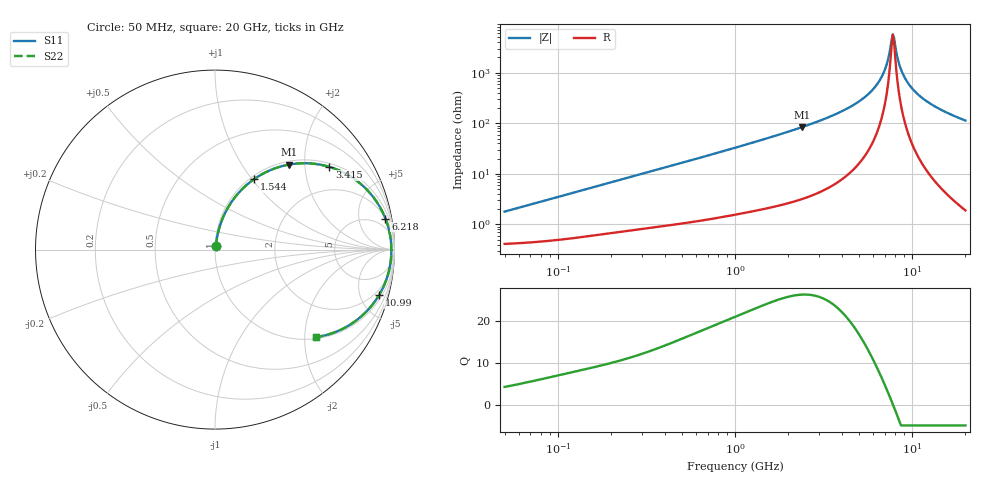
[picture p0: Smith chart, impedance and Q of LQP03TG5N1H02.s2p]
!Murata Part Number: LQP03TG5N1H02
!These Parameters are Measured in Series Mode Connection
!  o--[Z]--o
!Port1  Port2
!  o-------o
!Freq. Start=50[MHz] Stop=20[GHz], 401[Steps]
# Hz S RI R 50
!Freq.(Hz) S11(Real) S11(Imag) S21(Real) S21(Imag) S12(Real) S12(Imag) S22(Real) S22(Imag)
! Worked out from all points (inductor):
!   401 points, 50 MHz to 20 GHz, reference 50 ohm
!   read as one part in series: L = 5.55 nH near 51.52 MHz
!   highest Q = 26.4 at 2.384 GHz (marker M1), where L = 5.58 nH
!   self-resonance near 7.784 GHz
!   S11 on the Smith chart (normalised r, x): 50 MHz: 1.01, +0.03; 1.544 GHz: 1.04, +1.03; 3.415 GHz: 1.11, +2.68; 6.218 GHz: 2, +11; 10.99 GHz: 1.40, -7.03; 20 GHz: 1.04, -2.27
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5e7  0.00441 0.0173  0.9956 -0.0173  0.9956 -0.0173  0.00441 0.0173
1.364002e8  0.00775 0.0461  0.9922 -0.0461  0.9922 -0.0461  0.00775 0.0461
3.721004e8  0.0235 0.1192  0.9765 -0.1192  0.9765 -0.1192  0.0235 0.1192
1e9  0.1081 0.2877  0.8919 -0.2877  0.8919 -0.2877  0.1081 0.2877
1.544007e9  0.2184 0.3931  0.7816 -0.3931  0.7816 -0.3931  0.2184 0.3931
2.383959e9  0.4145 0.4741  0.5855 -0.4741  0.5855 -0.4741  0.4145 0.4741
2.728004e9  0.4936 0.4813  0.5064 -0.4813  0.5064 -0.4813  0.4936 0.4813
3.415248e9  0.6367 0.4611  0.3633 -0.4611  0.3633 -0.4611  0.6367 0.4611
4.89267e9  0.8531 0.3267  0.1469 -0.3267  0.1469 -0.3267  0.8531 0.3267
5.598765e9  0.9143 0.245  0.0857 -0.245  0.0857 -0.245  0.9143 0.245
6.217679e9  0.9497 0.1725  0.0503 -0.1725  0.0503 -0.1725  0.9497 0.1725
6.905011e9  0.9728 0.0945  0.0272 -0.0945  0.0272 -0.0945  0.9728 0.0945
7.222371e9  0.9786 0.0599  0.0214 -0.0599  0.0214 -0.0599  0.9786 0.0599
7.442007e9  0.9811 0.0366  0.0189 -0.0366  0.0189 -0.0366  0.9811 0.0366
7.668323e9  0.9825 0.0132  0.0175 -0.0132  0.0175 -0.0132  0.9825 0.0132
7.901521e9  0.9828 -0.0103  0.0172 0.0103  0.0172 0.0103  0.9828 -0.0103
8.389408e9  0.9799 -0.0571  0.0201 0.0571  0.0201 0.0571  0.9799 -0.0571
8.907419e9  0.9725 -0.1034  0.0275 0.1034  0.0275 0.1034  0.9725 -0.1034
9.745021e9  0.9533 -0.1709  0.0467 0.1709  0.0467 0.1709  0.9533 -0.1709
1.098561e10  0.9133 -0.2548  0.0867 0.2548  0.0867 0.2548  0.9133 -0.2548
1.417136e10  0.7841 -0.3969  0.2159 0.3969  0.2159 0.3969  0.7841 -0.3969
2e10  0.5613 -0.4879  0.4387 0.4879  0.4387 0.4879  0.5613 -0.4879
